(* Logix 5000 DataType export RTA_STRING_4096; software revision 32.00 *)

TYPE RTA_STRING_4096 :   // string type; String data type with up to 4096 characters available.
STRUCT
   LEN : DINT;
   DATA : SINT[4096];
END_STRUCT
END_TYPE
